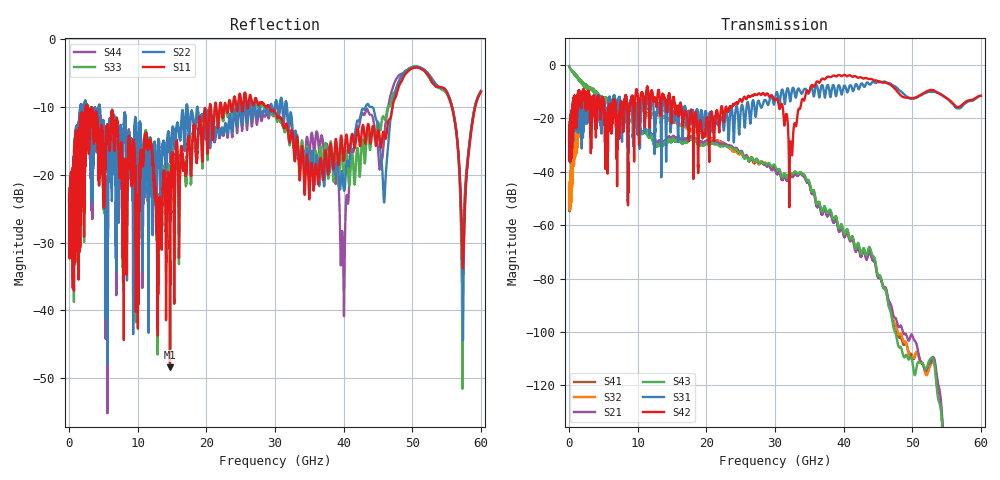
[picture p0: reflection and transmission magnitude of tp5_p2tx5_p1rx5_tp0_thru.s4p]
! 100G CR Analysis
! File: tp5_p2tx5_p1rx5_tp0_thru
! Description: 2m Cu Cable, OSFP, TP0-TP5
! Port Mapping
! Port1 -- P1RX5N
! Port2 -- P2TX5N
! Port3 -- P1RX5P
! Port4 -- P2TX5P
# GHz S MA R 50.00
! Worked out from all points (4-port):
!   6000 points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, 10 MHz to 60 GHz, reference 50 ohm
!   strongest paths, dB at 10 MHz, 15.01 GHz, 30.01 GHz, 45.01 GHz, 60 GHz:
!     S42: -28.0, -16.7, -13.2, -6.3, -11.6
!     S31: -27.9, -18.4, -12.9, -6.2, -11.6
!     S43: -0.5, -28.4, -37.7, -78.8, -171.6
!     S21: -0.5, -27.3, -39.3, -79.7, -190.4
!     S32: -46.1, -20.9, -38.2, -79.2, -183.7
!     S41: -46.3, -20.7, -38.7, -79.3, -177.1
!   lowest |S11| = -48.4 dB at 14.7 GHz (marker M1), VSWR 1.01, Z = 50.3 - j0.204 ohm
!   |S11| at or under -10 dB: 2.684 GHz to 20.48 GHz (17.8 GHz wide, 154 % of centre); 29.19 GHz to 47.12 GHz (17.93 GHz wide, 47 % of centre); 55.78 GHz to 59.17 GHz (3.39 GHz wide, 5.9 % of centre)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
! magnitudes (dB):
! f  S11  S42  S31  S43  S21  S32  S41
! 10 MHz  -24.0  -28.0  -27.9  -0.5  -0.5  -46.1  -46.3
! 2.92 GHz  -11.6  -11.2  -11.9  -9.4  -9.4  -14.5  -14.3
! 14.7 GHz  -48.4  -11.7  -20.5  -28.1  -27.0  -21.0  -20.8
! 39.86 GHz  -16.6  -4.0  -9.7  -61.2  -62.4  -62.0  -61.6
! 50.77 GHz  -4.2  -11.9  -12.1  -111.6  -106.0  -107.7  -107.7
! 57.33 GHz  -33.0  -14.7  -15.3  -162.8  -170.2  -161.6  -165.9
! 60 GHz  -7.7  -11.6  -11.6  -171.6  -190.4  -183.7  -177.1
